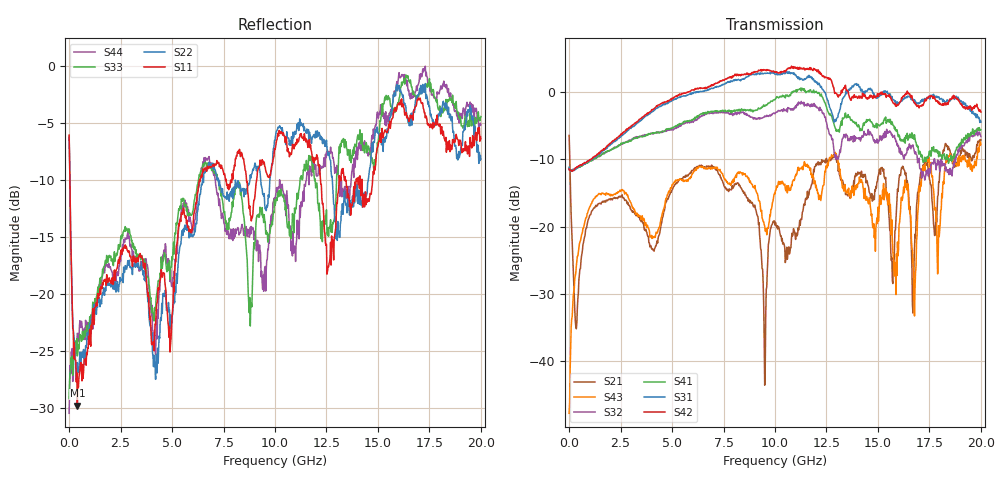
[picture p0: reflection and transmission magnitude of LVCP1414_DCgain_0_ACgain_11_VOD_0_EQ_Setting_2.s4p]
!Agilent Technologies,N5230A,MY46400459,A.07.50.48
!Agilent N5230A: A.07.50.48
!Date: Tuesday, April 17, 2012 18:37:29
!Correction: S11(Full 4 Port(1,2,3,4))
!S12(Full 4 Port(1,2,3,4))
!S13(Full 4 Port(1,2,3,4))
!S14(Full 4 Port(1,2,3,4))
!S21(Full 4 Port(1,2,3,4))
!S22(Full 4 Port(1,2,3,4))
!S23(Full 4 Port(1,2,3,4))
!S24(Full 4 Port(1,2,3,4))
!S31(Full 4 Port(1,2,3,4))
!S32(Full 4 Port(1,2,3,4))
!S33(Full 4 Port(1,2,3,4))
!S34(Full 4 Port(1,2,3,4))
!S41(Full 4 Port(1,2,3,4))
!S42(Full 4 Port(1,2,3,4))
!S43(Full 4 Port(1,2,3,4))
!S44(Full 4 Port(1,2,3,4))
!S4P File: Measurements: <S11,S12,S13,S14>,
!<S21,S22,S23,S24>,
!<S31,S32,S33,S34>,
!<S41,S42,S43,S44>:
# Hz S  dB  R 50
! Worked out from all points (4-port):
!   801 points, 300 kHz to 20 GHz, reference 50 ohm
!   strongest paths, dB at 300 kHz, 5 GHz, 10 GHz, 15 GHz, 20 GHz:
!     S42: -11.5, -0.9, 2.9, -0.4, -3.0
!     S31: -11.2, -1.3, 2.6, -0.8, -4.5
!     S41: -11.3, -5.3, -1.2, -4.9, -5.6
!     S32: -11.4, -5.6, -3.2, -7.6, -6.6
!     S43: -47.8, -13.8, -15.2, -17.1, -7.8
!     S21: -6.5, -14.6, -19.8, -12.6, -7.1
!   lowest |S11| = -29.8 dB at 400.3 MHz (marker M1), VSWR 1.07, Z = 53.1 + j1.36 ohm
!   |S11| at or under -10 dB: 37.72 MHz to 6.324 GHz (6.287 GHz wide, 198 % of centre); 12.21 GHz to 13.12 GHz (903.9 MHz wide, 7.14 % of centre); 13.42 GHz to 13.94 GHz (524.7 MHz wide, 3.84 % of centre)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
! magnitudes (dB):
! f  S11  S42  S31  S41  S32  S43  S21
! 300 kHz  -6.1  -11.5  -11.2  -11.3  -11.4  -47.8  -6.5
! 400.3 MHz  -29.8  -11.2  -11.1  -11.3  -11.2  -24.4  -32.1
! 1.55 GHz  -19.3  -8.8  -9.1  -9.5  -9.3  -15.3  -16.7
! 10.05 GHz  -6.8  2.9  2.6  -1.0  -3.0  -14.6  -19.7
! 12.7 GHz  -15.5  1.9  -2.7  -3.4  -6.5  -9.8  -10.2
! 16.78 GHz  -3.8  -1.6  -1.2  -6.4  -9.0  -33.3  -23.5
! 20 GHz  -6.4  -3.0  -4.5  -5.6  -6.6  -7.8  -7.1
